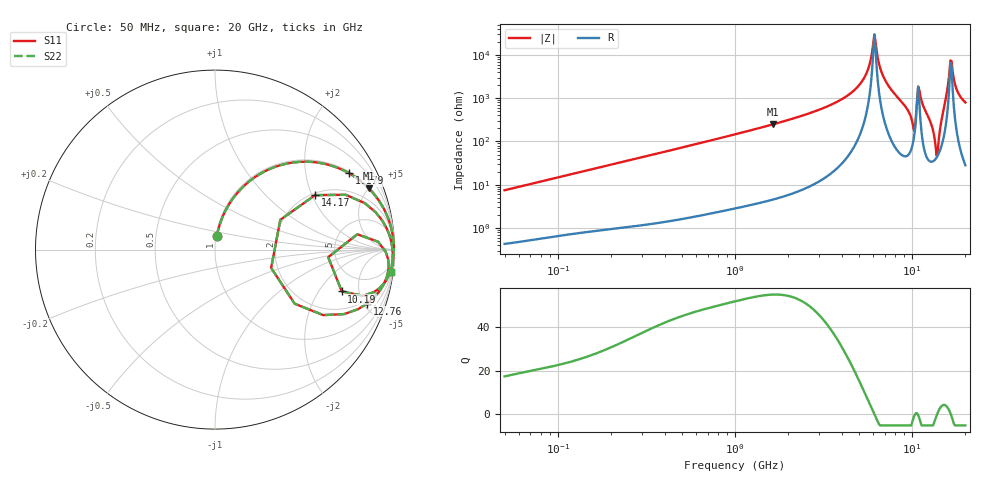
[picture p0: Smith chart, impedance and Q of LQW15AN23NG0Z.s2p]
!Murata Part Number: LQW15AN23NG0Z
!These Parameters are Measured in Series Mode Connection
!  o--[Z]--o
!Port1  Port2
!  o-------o
!Freq. Start=50[MHz] Stop=20[GHz], 401[Steps]
# Hz S RI R 50
!Freq.(Hz) S11(Real) S11(Imag) S21(Real) S21(Imag) S12(Real) S12(Imag) S22(Real) S22(Imag)
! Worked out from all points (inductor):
!   401 points, 50 MHz to 20 GHz, reference 50 ohm
!   read as one part in series: L = 23.7 nH near 51.52 MHz
!   highest Q = 54.6 at 1.639 GHz (marker M1), where L = 24.2 nH
!   self-resonance near 6.125 GHz
!   S11 on the Smith chart (normalised r, x): 50 MHz: 1.01, +0.15; 1.179 GHz: 1.07, +3.47; 10.19 GHz: 3.18, -3.32; 12.76 GHz: 1.68, -5.29; 14.17 GHz: 2.07, +2.11; 20 GHz: 2, -16
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5e7  0.00977 0.0737  0.9902 -0.0737  0.9902 -0.0737  0.00977 0.0737
1.364002e8  0.0452 0.189  0.9548 -0.189  0.9548 -0.189  0.0452 0.189
3.721004e8  0.2299 0.4087  0.7701 -0.4087  0.7701 -0.4087  0.2299 0.4087
1e9  0.6779 0.4577  0.3221 -0.4577  0.3221 -0.4577  0.6779 0.4577
1.179116e9  0.7472 0.4253  0.2528 -0.4253  0.2528 -0.4253  0.7472 0.4253
1.639343e9  0.8567 0.3414  0.1433 -0.3414  0.1433 -0.3414  0.8567 0.3414
2.728004e9  0.9534 0.2008  0.0466 -0.2008  0.0466 -0.2008  0.9534 0.2008
4.89267e9  0.9936 0.0557  0.00635 -0.0557  0.00635 -0.0557  0.9936 0.0557
5.515528e9  0.996 0.0266  0.00395 -0.0266  0.00395 -0.0266  0.996 0.0266
6.125241e9  0.9967 0.000321  0.00334 -0.000321  0.00334 -0.000321  0.9967 0.000321
6.701223e9  0.9959 -0.0236  0.00411 0.0236  0.00411 0.0236  0.9959 -0.0236
7.442007e9  0.9929 -0.0546  0.00708 0.0546  0.00708 0.0546  0.9929 -0.0546
9.457416e9  0.9509 -0.1755  0.0491 0.1755  0.0491 0.1755  0.9509 -0.1755
1.019291e10  0.7064 -0.233  0.2936 0.233  0.2936 0.233  0.7064 -0.233
1.098561e10  0.9642 -0.0514  0.0358 0.0514  0.0358 0.0514  0.9642 -0.0514
1.276073e10  0.8477 -0.3005  0.1523 0.3005  0.1523 0.3005  0.8477 -0.3005
1.334722e10  0.6034 -0.365  0.3966 0.365  0.3966 0.365  0.6034 -0.365
1.417136e10  0.5576 0.3035  0.4424 -0.3035  0.4424 -0.3035  0.5576 0.3035
1.504638e10  0.9319 0.162  0.0681 -0.162  0.0681 -0.162  0.9319 0.162
1.646126e10  0.9882 0.00614  0.0118 -0.00614  0.0118 -0.00614  0.9882 0.00614
1.828096e10  0.9881 -0.0759  0.0119 0.0759  0.0119 0.0759  0.9881 -0.0759
2e10  0.9803 -0.1225  0.0197 0.1225  0.0197 0.1225  0.9803 -0.1225
